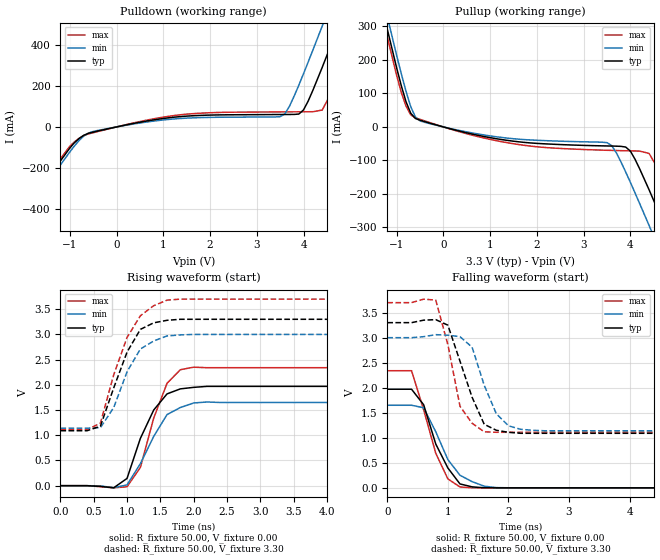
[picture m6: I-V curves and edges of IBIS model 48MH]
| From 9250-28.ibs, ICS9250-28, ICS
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|   Model 48MH
[Model]   48MH
Model_type   Output
Polarity   Non-Inverting
Vmeas = 1.5V
Cref = 20pF
Rref = 0
Vref = 1.5V
C_comp   5.50pF   5.00pF   6.00pF
[Temperature Range]   27.00   70.00   0.00
[Voltage Range]   3.30V   3.00V   3.70V
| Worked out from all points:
|   slope of the pulldown table from 0 to 0.495 V, typ, clamps not added: 21.7 ohm
|   slope of the pullup table from 0 to 0.495 V, typ, clamps not added: 28.3 ohm
|   rising waveform, R_fixture 50.00, V_fixture 0.00: 20-80 % time 385ps typ, 409ps min, 332ps max; typ from 0 V to 1.97 V
|   rising waveform, R_fixture 50.00, V_fixture 3.30: 20-80 % time 400ps typ, 383ps min, 432ps max; typ from 1.09 V to 3.3 V
|   falling waveform, R_fixture 50.00, V_fixture 0.00: 20-80 % time 380ps typ, 433ps min, 367ps max; typ from 1.97 V to 0 V
|   falling waveform, R_fixture 50.00, V_fixture 3.30: 20-80 % time 394ps typ, 341ps min, 274ps max; typ from 3.3 V to 1.09 V
[Pulldown]
| voltage   I(typ)   I(min)   I(max)
-3.3V     -857.6mA   -878.1mA   -844.8mA
-2.3V     -523.7mA   -544.6mA   -510.7mA
-2.1V     -457.3mA   -478.3mA   -444.3mA
-1V       -103.4mA   -122.4mA   -94.36mA
-600mV    -31.06mA   -29.9mA    -34.29mA
1.3V      49.19mA    40.27mA    57.7mA
3.5V      60.76mA    50.03mA    73.47mA
4V        83.02mA    260.4mA    74.12mA
4.4V      291.1mA    492.9mA    82.43mA
4.8V      525.9mA    731mA      280.2mA
5.2V      765.3mA    971.6mA    515.2mA
6.2V      1.37A      1.58A      1.12A
[Pullup]
| voltage   I(typ)   I(min)   I(max)
-3.3V     1.55A      1.58A      1.53A
-1.5V     464.7mA    502.9mA    441mA
-1V       175.9mA    213.2mA    153.4mA
-800mV    75.17mA    106.3mA    62.05mA
-600mV    25.23mA    29.87mA    27.35mA
1.4V      -40.8mA    -33.83mA   -47.88mA
3.5V      -56.8mA    -46.99mA   -69.7mA
4V        -72.19mA   -165.5mA   -71.39mA
4.4V      -187.6mA   -294.1mA   -79.04mA
4.8V      -317.5mA   -425.8mA   -188.7mA
5.2V      -449.9mA   -558.8mA   -318.7mA
6.2V      -784.7mA   -893.8mA   -652.2mA
[Ramp]
| variable   typ   min   max
dV/dt_r   1.18/286.75p   991.20m/325.25p   1.41/260.12p
dV/dt_f   1.32/300.00p   1.12/300.00p   1.55/300.00p
[Rising Waveform]
R_fixture = 50.00
V_fixture = 0.00
V_fixture_min = 0.00
V_fixture_max = 0.00
| time   V(typ)   V(min)   V(max)
0s        0V         0V         0V
600ps     -14.46mV   -4.31mV    -20.2mV
800ps     -41.42mV   -40.89mV   -43.25mV
1ns       144.3mV    15.76mV    -20.58mV
1.2ns     937.9mV    436.2mV    361.8mV
1.4ns     1.5V       976.3mV    1.34V
1.6ns     1.82V      1.41V      2.03V
1.8ns     1.92V      1.55V      2.3V
2ns       1.95V      1.64V      2.35V
10ns      1.97V      1.65V      2.34V
[Rising Waveform]
R_fixture = 50.00
V_fixture = 3.30
V_fixture_min = 3.00
V_fixture_max = 3.70
| time   V(typ)   V(min)   V(max)
0s        1.09V      1.14V      1.11V
400ps     1.09V      1.14V      1.11V
600ps     1.18V      1.15V      1.24V
800ps     1.94V      1.55V      2.2V
1ns       2.65V      2.26V      2.94V
1.2ns     3.1V       2.71V      3.37V
1.4ns     3.23V      2.87V      3.57V
1.6ns     3.28V      2.97V      3.68V
2ns       3.3V       3V         3.7V
10ns      3.3V       3V         3.7V
[Falling Waveform]
R_fixture = 50.00
V_fixture = 0.00
V_fixture_min = 0.00
V_fixture_max = 0.00
| time   V(typ)   V(min)   V(max)
0s        1.97V      1.65V      2.34V
400ps     1.97V      1.65V      2.34V
600ps     1.66V      1.6V       1.56V
800ps     875mV      1.12V      690.9mV
1ns       396.8mV    563.8mV    178mV
1.2ns     77.74mV    251.5mV    17.85mV
1.4ns     19.93mV    124mV      343.7uV
1.6ns     1.31mV     33.34mV    152.5uV
1.8ns     303.3uV    5.09mV     10.5uV
10ns      -815.8nV   -5.53uV    -4.46uV
[Falling Waveform]
R_fixture = 50.00
V_fixture = 3.30
V_fixture_min = 3.00
V_fixture_max = 3.70
| time   V(typ)   V(min)   V(max)
0s        3.3V       3V         3.7V
800ps     3.36V      3.06V      3.75V
1ns       3.25V      3.05V      2.86V
1.2ns     2.53V      3.02V      1.63V
1.4ns     1.81V      2.81V      1.29V
1.6ns     1.27V      2.05V      1.12V
1.8ns     1.15V      1.48V      1.11V
2ns       1.11V      1.24V      1.11V
2.2ns     1.09V      1.17V      1.11V
10ns      1.09V      1.14V      1.11V
